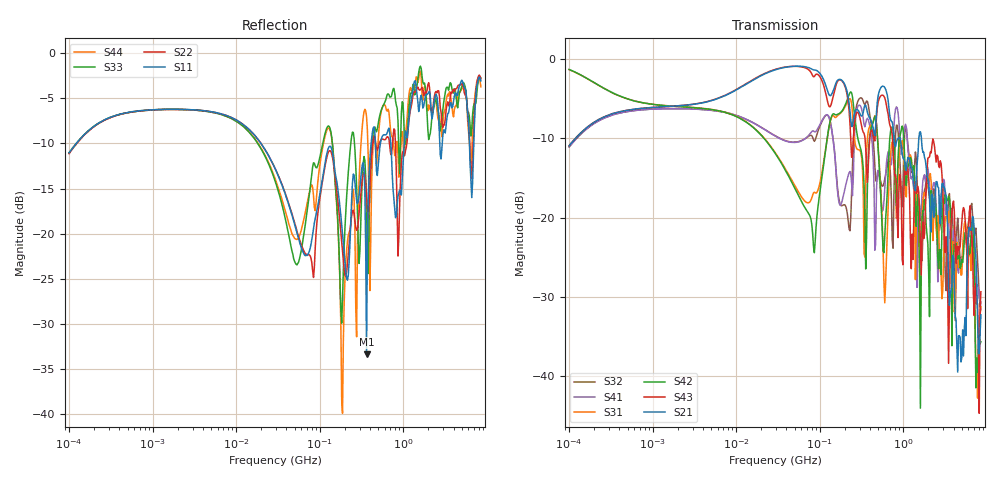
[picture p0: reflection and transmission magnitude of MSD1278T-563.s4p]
# MHz S MA R 50
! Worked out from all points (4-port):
!   498 points, 100 kHz to 8.5 GHz, reference 50 ohm
!   strongest paths, dB at 100 kHz, 1.698 MHz, 29.49 MHz, 500.7 MHz, 8.5 GHz:
!     S21: -11.0, -6.0, -1.4, -4.6, -32.3
!     S43: -10.9, -6.0, -1.3, -5.5, -29.3
!     S42: -1.3, -5.9, -11.9, -11.3, -35.6
!     S31: -1.3, -5.9, -11.9, -11.0, -31.2
!     S41: -11.1, -6.3, -9.7, -14.0, -31.6
!     S32: -11.1, -6.3, -9.7, -14.5, -30.6
!   lowest |S11| = -33.4 dB at 363.7 MHz (marker M1), VSWR 1.04, Z = 51.4 + j1.7 ohm
!   |S11| at or under -10 dB: 19.79 MHz to 412.7 MHz (392.9 MHz wide, 182 % of centre); 709 MHz to 1.03 GHz (320.7 MHz wide, 36.9 % of centre); 6.199 GHz to 6.997 GHz (797.6 MHz wide, 12.1 % of centre)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
0.1  0.2809 52.9  0.2831 54.0  0.8574 -15.6  0.2791 -126.8
     0.2831 54.0  0.2776 53.1  0.2789 -126.7  0.8585 -15.6
     0.8574 -15.6  0.2789 -126.7  0.2802 53.1  0.2837 53.9
     0.2791 -126.8  0.8585 -15.6  0.2837 53.9  0.2798 53.5
127.1871  0.2982 -28.5  0.6067 -38.8  0.3552 125.2  0.4365 -0.5
          0.6067 -38.8  0.2835 -33.0  0.4361 -1.4  0.3562 120.1
          0.3552 125.2  0.4361 -1.4  0.3955 -24.0  0.5145 -45.1
          0.4365 -0.5  0.3562 120.1  0.5145 -45.1  0.3853 -29.3
187.5231  0.1007 -127.9  0.7266 -49.3  0.4698 34.5  0.1303 7.6
          0.7266 -49.3  0.07837 -159.2  0.1193 -6.0  0.4754 30.7
          0.4698 34.5  0.1193 -6.0  0.04329 17.4  0.7203 -58.7
          0.1303 7.6  0.4754 30.7  0.7203 -58.7  0.01012 11.7
363.6528  0.02149 50.5  0.4868 -64.4  0.2572 13.5  0.416 -42.1
          0.4868 -64.4  0.165 39.2  0.5438 -42.1  0.074 77.0
          0.2572 13.5  0.5438 -42.1  0.1385 -66.8  0.2022 -85.9
          0.416 -42.1  0.074 77.0  0.2022 -85.9  0.445 -32.5
1604.647  0.5647 -140.8  0.3475 170.5  0.02342 173.1  0.09591 -159.6
          0.3475 170.5  0.6281 -138.9  0.06032 165.6  0.006284 -118.1
          0.02342 173.1  0.06032 165.6  0.8478 -150.8  0.07002 148.1
          0.09591 -159.6  0.006284 -118.1  0.07002 148.1  0.7955 -153.9
3183.684  0.3617 76.5  0.1455 -87.0  0.1013 61.6  0.1137 14.3
          0.1455 -87.0  0.4309 70.7  0.04339 18.0  0.1394 53.8
          0.1013 61.6  0.04339 18.0  0.6044 70.7  0.06021 -36.7
          0.1137 14.3  0.1394 53.8  0.06021 -36.7  0.4915 64.1
8500  0.7021 -54.1  0.02437 -37.3  0.02739 -68.8  0.02623 -173.9
      0.02437 -37.3  0.7219 -55.2  0.02935 -132.2  0.01651 -77.8
      0.02739 -68.8  0.02935 -132.2  0.7291 -54.7  0.03408 -37.9
      0.02623 -173.9  0.01651 -77.8  0.03408 -37.9  0.6518 -56.6
